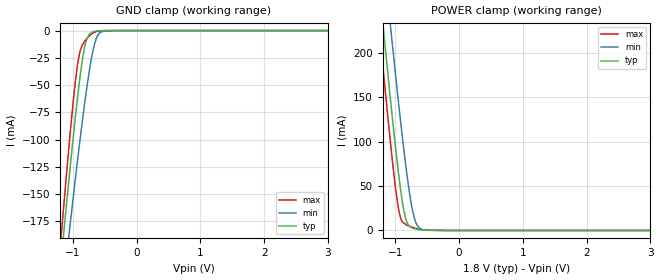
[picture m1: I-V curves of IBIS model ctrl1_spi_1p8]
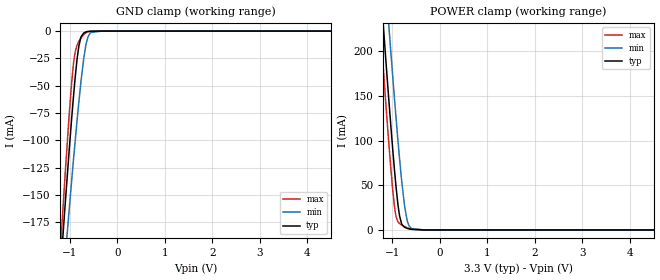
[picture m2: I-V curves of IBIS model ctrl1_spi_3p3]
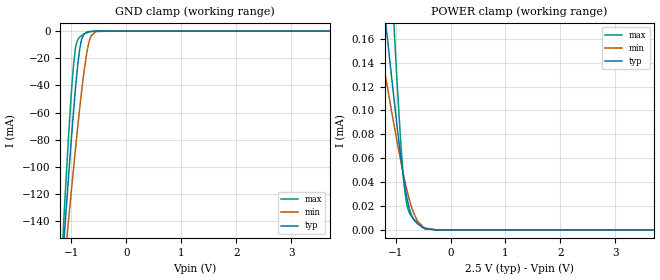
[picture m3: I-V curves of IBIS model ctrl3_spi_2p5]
|Texas Instruments Incorporated
| FPC401 Quad Port Controller
| Marketing part#   Digital Voltage Range   Package-type   #pins
| FPC401   1.65V-3.6V   QFN   56
[IBIS Ver]   4.1
[File name]   fpc401.ibs
[File Rev]   1.0
[Date]   7/15/2016
[Source]
| Texas Instruments Incorporated.
| Analog-eLab Design Center, HPA
| 12500 TI Blvd
| Dallas, TX -75243
[Notes]   Revision History:
| Rev 1.0: 7/15/2016
| - Initial version of the model
| - Model generated from simulations in SPECTRE
| - Model matched to SPICE simulation
| - C_comp although listed in numerical order of value are
|   obtained from varying PVT conditions. For PVT conditions for
|   each specific value refer the buffer description under
|   respective [Model]. IBIS model user is responsible for using
|   appropriate C_comp to simulate for Signal Integrity.
[Disclaimer]
| This model is designed as an aid for customers of Texas Instruments.
| TI and its licensors and suppliers make no warranties, either expressed
| or implied, with respect to this  model, including the warranties of
| merchantability or fitness for a particular purpose. The model is
| provided solely on an "as is" basis. The entire risk as to its quality
| and performance is with the customer.
[Copyright]
(C) Copyright 2016 Texas Instruments Incorporated.All rights reserved.
|   FPC401
[Component]   FPC401
[Manufacturer]   TI
[Package]   |56 QFN
|   typ   min   max
R_pkg   0.067   0.027   0.083
L_pkg   0.937nH   0.593nH   1.143nH
C_pkg   0.144pF   0.126pF   0.200pF
[Pin]  signal_name   model_name   R_pin   L_pin   C_pin
1   IN_B[2]   in_a0   na   na   na
2   OUT_B[2]   out_a0   na   na   na
3   IN_C[2]   in_a0   na   na   na
4   MOD_SCL[2]   mod_scl0   na   na   na
5   MOD_SDA[2]   mod_scl0   na   na   na
6   OUT_C[2]   out_c0   na   na   na
7   OUT_D[2]   out_c0   na   na   na
8   GPIO[2]   gpio3   na   na   na
9   VDD1   power   na   na   na
10   IN_A[3]   in_a0   na   na   na
11   OUT_A[3]   out_a0   na   na   na
12   IN_B[3]   in_a0   na   na   na
13   OUT_B[3]   out_a0   na   na   na
14   IN_C[3]   in_c3   na   na   na
15   MOD_SCL[3]   mod_scl0   na   na   na
16   MOD_SDA[3]   mod_scl0   na   na   na
17   OUT_C[3]   out_c0   na   na   na
18   OUT_D[3]   out_c0   na   na   na
19   GPIO[3]   gpio3   na   na   na
20   VDD2   power   na   na   na
21   CTRL4   ctrl4   na   na   na
22   EN   ctrl3   na   na   na
23   CTRL1   ctrl1   na   na   na
24   CTRL2   ctrl1   na   na   na
25   HOST_INT_N   host_int_n   na   na   na
26   VDD2   power   na   na   na
27   GND   power   na   na   na
28   CTRL3   ctrl3   na   na   na
29   TEST_N   test_n   na   na   na
30   SPI_LED_SYNC   spi_led_sync   na   na   na
31   PROTOCOL_SEL   in_a0   na   na   na
32   CAPL   nc   na   na   na
33   OUT_D[0]   out_c0   na   na   na
34   OUT_C[0]   out_c0   na   na   na
35   MOD_SDA[0]   mod_scl0   na   na   na
36   MOD_SCL[0]   mod_scl0   na   na   na
37   IN_C[0]   in_a0   na   na   na
38   OUT_B[0]   out_a0   na   na   na
39   IN_B[0]   in_a0   na   na   na
40   OUT_A[0]   out_a0   na   na   na
41   IN_A[0]   in_a0   na   na   na
42   GPIO[0]   gpio1   na   na   na
43   VDD1   power   na   na   na
44   OUT_A[1]   out_a0   na   na   na
45   OUT_B[1]   out_a0   na   na   na
46   IN_C[1]   in_a0   na   na   na
47   IN_B[1]   in_a0   na   na   na
48   MOD_SDA[1]   mod_scl0   na   na   na
49   MOD_SCL[1]   mod_scl0   na   na   na
50   IN_A[1]   in_a0   na   na   na
51   OUT_C[1]   out_c0   na   na   na
52   OUT_D[1]   out_c0   na   na   na
53   GPIO[1]   gpio1   na   na   na
54   VDD1   power   na   na   na
55   IN_A[2]   in_a0   na   na   na
56   OUT_A[2]   out_a0   na   na   na
|   Model Selectors
[Model Selector] ctrl1
ctrl1_spi_1p8   1.8  digital Input
ctrl1_spi_2p5   2.5  digital Input
ctrl1_spi_3p3   3.3  digital Input
ctrl1_i2c_1p8   1.8  digital I/O_open_drain
ctrl1_i2c_2p5   2.5  digital I/O_open_drain
ctrl1_i2c_3p3   3.3  digital I/O_open_drain
[Model Selector] ctrl3
ctrl3_spi_1p8   1.8  digital Input
ctrl3_spi_2p5   2.5  digital Input
ctrl3_spi_3p3   3.3  digital Input
[Model Selector] ctrl4
ctrl4_spi_1p8   1.8  digital Output
ctrl4_spi_2p5   2.5  digital Output
ctrl4_spi_3p3   3.3  digital Output
ctrl4_i2c_1p8   1.8  digital I/O_open_drain
ctrl4_i2c_2p5   2.5  digital I/O_open_drain
ctrl4_i2c_3p3   3.3  digital I/O_open_drain
[Model Selector] host_int_n
host_int_n_1p8   1.8   digital I/O_open_drain
host_int_n_2p5   2.5   digital I/O_open_drain
host_int_n_3p3   3.3   digital I/O_open_drain
| Models and submodels in the file (27): ctrl1_spi_1p8 (Input), ctrl1_spi_2p5 (Input), ctrl1_spi_3p3 (Input), ctrl3_spi_1p8 (Input), ctrl3_spi_2p5 (Input), ctrl3_spi_3p3 (Input), in_a0 (Input), in_c3 (Input), test_n (Input), ctrl4_spi_1p8 (Output), ctrl4_spi_2p5 (Output), ctrl4_spi_3p3 (Output), out_a0 (Output), out_c0 (Output), ctrl4_i2c_1p8 (I/O_open_drain), ctrl4_i2c_2p5 (I/O_open_drain), ctrl4_i2c_3p3 (I/O_open_drain), gpio1 (I/O), gpio3 (I/O), mod_scl0 (I/O_open_drain), spi_led_sync (I/O), ctrl1_i2c_1p8 (I/O_open_drain), ctrl1_i2c_2p5 (I/O_open_drain), ctrl1_i2c_3p3 (I/O_open_drain), host_int_n_1p8 (I/O_open_drain), host_int_n_2p5 (I/O_open_drain), host_int_n_3p3 (I/O_open_drain)
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|   ctrl1_spi_1p8 Model
[Model]   ctrl1_spi_1p8
Model_type   Input
Vinl = 0.54
Vinh = 1.26
|   typ   min   max
|   (nom PVT)   (fast PVT)   (slow PVT)
C_comp   3.494e-12   3.459e-12   3.529e-12
| Where nom  PVT is Nominal Process, 1.8V, 27C
|   Fast PVT is Strong Process,  1.95V, -40C
|   Slow PVT is Weak Process,   1.65V, 125C
[Voltage Range]   1.8   1.65   1.95
|Junction Temperature
[Temperature Range]   27   125   -40
[Power Clamp Reference]   1.8   1.65   1.95
[GND Clamp Reference]   0   0   0
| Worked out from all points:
|   GND clamp passes 1 mA (typ) near -0.68 V on its own axis
|   POWER clamp passes 1 mA (typ) near -0.63 V on its own axis
[GND Clamp]
|   Voltage   I(typ)   I(min)   I(max)
-1.8V     -607.7mA   -595.9mA   -640.8mA
-1.191V   -214.8mA   -256.5mA   -193.9mA
-1.151V   -189.9mA   -234.7mA   -165.8mA
-1.048V   -128.1mA   -180.3mA   -97.16mA
-971.2mV  -84.77mA   -141.2mA   -51.83mA
-926.4mV  -60.99mA   -118.8mA   -30.81mA
-885.6mV  -41.21mA   -99.01mA   -18.64mA
-815.4mV  -14.86mA   -66.67mA   -9.798mA
-706mV    -1.675mA   -24.3mA    -3.051mA
-626.9mV  -378.7uA   -6.237mA   -804.6uA
-499.8mV  -24.3uA    -228.5uA   -40.78uA
3.6V      0A         0A         0A
[POWER Clamp]
|   Voltage   I(typ)   I(min)   I(max)
-1.8V     697.6mA    770.2mA    663mA
-1.409V   393mA      472.9mA    349.1mA
-1.208V   241.5mA    324.2mA    193.7mA
-1.17V    213.8mA    296.7mA    165.4mA
-1.073V   144.3mA    227.3mA    95.64mA
-952.2mV  65.14mA    144.7mA    24.89mA
-901.1mV  37.02mA    111.6mA    11.21mA
-838mV    13.02mA    73.48mA    6.749mA
-757.8mV  3.491mA    32.76mA    4.193mA
-706mV    2.119mA    14.73mA    2.878mA
-563.7mV  440.1uA    785.5uA    538.9uA
3.6V      0A         0A         0A
|   ctrl1_spi_3p3 Model
[Model]   ctrl1_spi_3p3
Model_type   Input
Vinl = 0.99
Vinh = 2.31
|   typ   min   max
|   (nom PVT)   (fast PVT)   (slow PVT)
C_comp   3.611e-12   3.611e-12   3.611e-12
| Where nom  PVT is Nominal Process, 3.3V, 27C
|   Fast PVT is Strong Process,  3.6V, -40C
|   Slow PVT is Weak Process,   3V, 125C
[Voltage Range]   3.3   3   3.6
|Junction Temperature
[Temperature Range]   27   125   -40
[Power Clamp Reference]   3.3   3   3.6
[GND Clamp Reference]   0   0   0
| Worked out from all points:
|   GND clamp passes 1 mA (typ) near -0.68 V on its own axis
|   POWER clamp passes 1 mA (typ) near -0.63 V on its own axis
[GND Clamp]
|   Voltage   I(typ)   I(min)   I(max)
-3.3V     -1.62A     -1.468A    -1.788A
-1.266V   -260.5mA   -296.3mA   -245.6mA
-1.122V   -171.5mA   -218.7mA   -145.1mA
-1.083V   -148.1mA   -198.1mA   -119mA
-1.014V   -107.8mA   -162.3mA   -75.29mA
-904.2mV  -49.22mA   -107.3mA   -22.79mA
-811.8mV  -13.51mA   -64.5mA    -9.369mA
-765.6mV  -5.255mA   -45.18mA   -6.088mA
-663.3mV  -739.7uA   -12.46mA   -1.535mA
-564mV    -100.1uA   -1.281mA   -195.5uA
-330mV    -250.3nA   -2.129uA   -158.7nA
6.6V      0A         0A         0A
[POWER Clamp]
|   Voltage   I(typ)   I(min)   I(max)
-3.3V     1.909A     1.948A     1.91A
-1.267V   284.5mA    366.7mA    237.6mA
-1.147V   196.1mA    279.3mA    147.4mA
-1.083V   150.4mA    233.6mA    101.5mA
-1.036V   117.7mA    200.4mA    69.75mA
-993.3mV  89.76mA    171.4mA    44.17mA
-933.9mV  53.64mA    131.8mA    17.86mA
-848.1mV  15.33mA    78.5mA     7.091mA
-744mV    2.966mA    26.64mA    3.777mA
-646.8mV  1.205mA    4.293mA    1.631mA
-330mV    2.194uA    7.269uA    1.05uA
6.6V      0A         0A         0A
|   ctrl3_spi_2p5 Model
[Model]   ctrl3_spi_2p5
Model_type   Input
Vinl = 0.75
Vinh = 1.75
|   typ   min   max
|   (nom PVT)   (fast PVT)   (slow PVT)
C_comp   1.117e-12   1.115e-12   1.124e-12
| Where nom  PVT is Nominal Process, 2.5V, 27C
|   Fast PVT is Strong Process,  2.65V, -40C
|   Slow PVT is Weak Process,   2.35V, 125C
[Voltage Range]   2.5   2.35   2.65
|Junction Temperature
[Temperature Range]   27   125   -40
[Power Clamp Reference]   2.5   2.35   2.65
[GND Clamp Reference]   0   0   0
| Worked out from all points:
|   GND clamp passes 1 mA (typ) near -0.73 V on its own axis
[GND Clamp]
|   Voltage   I(typ)   I(min)   I(max)
-2.5V     -993.6mA   -802.3mA   -1.232A
-1.244V   -217.3mA   -222.9mA   -218.3mA
-1.133V   -152.1mA   -173.7mA   -134.3mA
-1.082V   -123.5mA   -151.9mA   -98.14mA
-1.05V    -105.9mA   -138.3mA   -76.3mA
-986.9mV  -71.83mA   -111.4mA   -37.23mA
-931.2mV  -44.5mA    -88.59mA   -13.94mA
-826.8mV  -8.299mA   -48.57mA   -3.652mA
-723.4mV  -793.8uA   -16.72mA   -1.304mA
-641.1mV  -173.8uA   -3.467mA   -363.6uA
-551.8mV  -28.02uA   -327.9uA   -52.76uA
5V        0A         0A         0A
[POWER Clamp]
|   Voltage   I(typ)   I(min)   I(max)
-2.5V     779.1uA    497.7uA    1.566mA
-1.356V   250.9uA    175uA      466.8uA
-1.196V   180.6uA    131.8uA    319uA
-1.062V   123uA      96.37uA    198.3uA
-978.9mV  89.04uA    75.29uA    128uA
-910mV    62.6uA     58.54uA    75.54uA
-870.2mV  48.63uA    49.34uA    50.51uA
-798.7mV  27.77uA    34.16uA    22.1uA
-684.7mV  9.819uA    15.8uA     9.906uA
-605.2mV  5.334uA    7.859uA    5.938uA
-462.6mV  1.064uA    1.632uA    983.7nA
5V        0A         0A         0A
